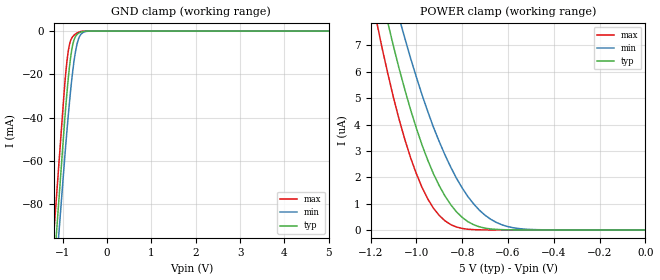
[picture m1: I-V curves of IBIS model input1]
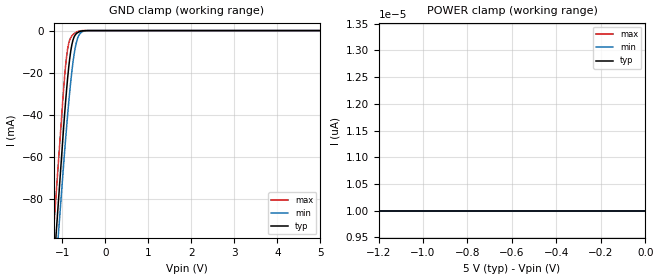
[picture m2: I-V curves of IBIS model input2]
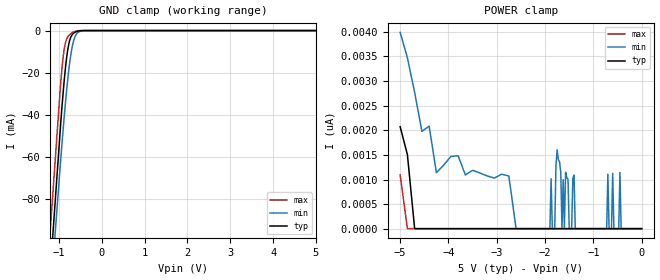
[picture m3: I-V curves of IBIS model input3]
|   Microchip Technology Inc.
|   93AA86C - 16 Kbit Microwire serial EEPROM
|   (Vcc = +1.8V to +5.5V)
|   150K Process
|   Copyright (C) 2018 Microchip Technology Inc.
[IBIS ver]   3.2
[File name]   93aa86c-i_st-5v.ibs
[File Rev]   1.0
[Date]   May 18, 2018
[Source]   Waveforms generated by SPICE simulation at Microchip.
   All other data taken from lab measurements at Microchip.
[Notes]   This IBIS model is for the Microchip 93AA86C device, a
   16 Kbit Microwire bus serial EEPROM manufactured on
   Microchip's 150K process, for industrial temp in a
   4.4 mm, 8-lead TSSOP package operating at 5V.
[Disclaimer] Unauthorized reproduction and/or distribution is
   strictly restricted. All rights reserved.
   This information is provided to you for your convenience
   and use with Microchip products only. Microchip
   disclaims all liability arising from this information
   and its use.
   THIS INFORMATION IS PROVIDED "AS IS." MICROCHIP MAKES NO
   REPRESENTATION OR WARRANTIES OF ANY KIND WHETHER EXPRESS
   OR IMPLIED, WRITTEN OR ORAL, STATUTORY OR OTHERWISE,
   RELATED TO THE INFORMATION PROVIDED TO YOU, INCLUDING
   BUT NOT LIMITED TO ITS CONDITION, QUALITY, PERFORMANCE,
   MERCHANTABILITY, NON-INFRINGEMENT, OR FITNESS FOR
   PURPOSE. MICROCHIP IS NOT LIABLE, UNDER ANY
   CIRCUMSTANCES, FOR SPECIAL, INCIDENTAL OR CONSEQUENTIAL
   DAMAGES, FOR ANY REASON WHATSOEVER.
   It is your responsibility to ensure that your
   application meets with your specifications.
|   Component 93AA86C-I/ST
[Component]   93AA86C-I/ST
[Manufacturer]   Microchip Technology Inc.
[Package]
| variable   typ   min   max
R_pkg   99.09m   85.92m   112.26m
L_pkg   2.16nH   1.55nH   2.76nH
C_pkg   0.49pF   0.43pF   0.55pF
[Pin]  signal_name   model_name
1   CS   input1
2   CLK   input2
3   DI   input3
4   DO   driver
5   VSS   GND
6   ORG   input4
7   PE   input5
8   VCC   POWER
| Models and submodels in the file (6): input1 (Input), input2 (Input), input3 (Input), driver (3-state), input4 (Input), input5 (Input)
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|   Model input1
[Model]   input1
Model_type   Input
Vinl = 0.8
Vinh = 2.0
C_comp   5.00pF   5.00pF   5.00pF
[Temperature Range]   25.00   85.00   -40.00
[Voltage Range]   5.00V   1.80V   5.50V
[Pullup Reference]   5.00V   5.00V   5.00V
[POWER Clamp Reference]   5.00V   5.00V   5.00V
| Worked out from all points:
|   GND clamp passes 1 mA (typ) near -0.64 V on its own axis
[GND_clamp]
| voltage   I(typ)   I(min)   I(max)
-5V       -1.185A    -1.135A    -1.164A
-1.25V    -124.7mA   -137.3mA   -107.7mA
-1.1V     -82.25mA   -97.41mA   -65.49mA
-1V       -53.97mA   -70.81mA   -37.33mA
-950mV    -40.03mA   -57.57mA   -23.76mA
-875mV    -22.02mA   -39.23mA   -9.343mA
-775mV    -6.431mA   -18.79mA   -2.594mA
-725mV    -3.025mA   -11.17mA   -1.545mA
-650mV    -1.099mA   -4.033mA   -587.6uA
-550mV    -229.9uA   -775.5uA   -60.37uA
-400mV    -2.588uA   -34.77uA   -111.3nA
5V        10pA       10pA       10pA
[POWER_clamp]
| voltage   I(typ)   I(min)   I(max)
-5V       24.92uA    20.24uA    30.57uA
-1.175V   9.818uA    11.45uA    7.976uA
-1.15V    8.826uA    10.56uA    6.925uA
-1.125V   7.889uA    9.713uA    5.956uA
-1.075V   6.121uA    8.049uA    4.192uA
-1.05V    5.317uA    7.268uA    3.428uA
-1V       3.866uA    5.805uA    2.138uA
-925mV    2.126uA    3.894uA    823.5nA
-825mV    689.9nA    1.966uA    111.9nA
-700mV    69.34nA    558.2nA    2.493nA
-550mV    1.499nA    50.52nA    10pA
0V        10pA       10pA       10pA
|   Model input2
[Model]   input2
Model_type   Input
Vinl = 0.8
Vinh = 2.0
C_comp   5.00pF   5.00pF   5.00pF
[Temperature Range]   25.00   85.00   -40.00
[Voltage Range]   5.00V   1.80V   5.50V
[Pullup Reference]   5.00V   5.00V   5.00V
[POWER Clamp Reference]   5.00V   5.00V   5.00V
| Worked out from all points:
|   GND clamp passes 1 mA (typ) near -0.64 V on its own axis
[GND_clamp]
| voltage   I(typ)   I(min)   I(max)
-5V       -1.223A    -1.168A    -1.194A
-1.25V    -129.2mA   -141.6mA   -110mA
-1.1V     -85.41mA   -100.6mA   -66.57mA
-1V       -56.25mA   -73.24mA   -37.65mA
-950mV    -41.88mA   -59.63mA   -23.72mA
-875mV    -23.22mA   -40.75mA   -9.1mA
-775mV    -6.823mA   -19.63mA   -2.548mA
-725mV    -3.166mA   -11.7mA    -1.52mA
-650mV    -1.126mA   -4.205mA   -569.7uA
-550mV    -237.5uA   -790.7uA   -55.38uA
-400mV    -2.822uA   -35.47uA   -92.42nA
5V        10pA       10pA       10pA
[POWER_clamp]
| voltage   I(typ)   I(min)   I(max)
-5V       1.163nA    2.944nA    10pA
-4.85V    10pA       2.361nA    10pA
-3.8V     10pA       1.005nA    10pA
-3.65V    10pA       10pA       10pA
0V        10pA       10pA       10pA
|   Model input3
[Model]   input3
Model_type   Input
Vinl = 0.8
Vinh = 2.0
C_comp   5.00pF   5.00pF   5.00pF
[Temperature Range]   25.00   85.00   -40.00
[Voltage Range]   5.00V   1.80V   5.50V
[Pullup Reference]   5.00V   5.00V   5.00V
[POWER Clamp Reference]   5.00V   5.00V   5.00V
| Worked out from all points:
|   GND clamp passes 1 mA (typ) near -0.64 V on its own axis
[GND_clamp]
| voltage   I(typ)   I(min)   I(max)
-5V       -1.21A     -1.15A     -1.186A
-1.25V    -128.6mA   -140.3mA   -108.9mA
-1.1V     -85.37mA   -99.89mA   -65.78mA
-950mV    -42.29mA   -59.57mA   -23.23mA
-900mV    -29.54mA   -47.02mA   -12.65mA
-850mV    -18.52mA   -35.22mA   -6.148mA
-775mV    -7.106mA   -19.99mA   -2.516mA
-725mV    -3.304mA   -12.03mA   -1.503mA
-650mV    -1.161mA   -4.394mA   -560.5uA
-550mV    -248.8uA   -830uA     -53.39uA
-400mV    -3.169uA   -38.35uA   -85.84nA
5V        10pA       10pA       10pA
[POWER_clamp]
| voltage   I(typ)   I(min)   I(max)
-5V       2.074nA    3.984nA    1.096nA
-4.7V     10pA       2.768nA    10pA
-4.25V    10pA       1.144nA    10pA
-1.8V     10pA       10pA       10pA
-1.75V    10pA       1.606nA    10pA
-1.65V    10pA       10pA       10pA
-1.575V   10pA       1.153nA    10pA
-1.5V     10pA       10pA       10pA
-600mV    10pA       1.128nA    10pA
-475mV    10pA       10pA       10pA
-450mV    10pA       1.149nA    10pA
0V        10pA       10pA       10pA
